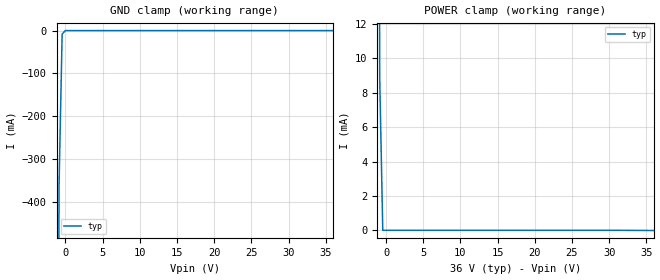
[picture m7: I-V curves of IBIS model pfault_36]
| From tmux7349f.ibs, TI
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| pfault_36
[Model]   pfault_36
Model_type   Input
Vinl = 0.8
Vinh = 1.3
|   typ   min   max
C_comp   1.008417e-11   NA   NA
[Voltage Range]   36   NA   NA
[Temperature Range]   27   NA   NA
[Power Clamp Reference]   36   NA   NA
[GND Clamp Reference]   0   NA   NA
[GND Clamp]
|   Voltage   I(typ)   I(min)   I(max)
-5V       -27.52A    NA         NA
-1.273V   -2.381A    NA         NA
-858.6mV  -359.2mA   NA         NA
-444.4mV  -8.401mA   NA         NA
-30.3mV   -18.71nA   NA         NA
36V       10.01uA    NA         NA
[POWER Clamp]
|   Voltage   I(typ)   I(min)   I(max)
-5V       1.413A     NA         NA
-1.273V   125.5mA    NA         NA
-858.6mV  8.928mA    NA         NA
-444.4mV  10.02uA    NA         NA
36V       -614.9pA   NA         NA
